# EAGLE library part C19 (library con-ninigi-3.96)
NINIGI
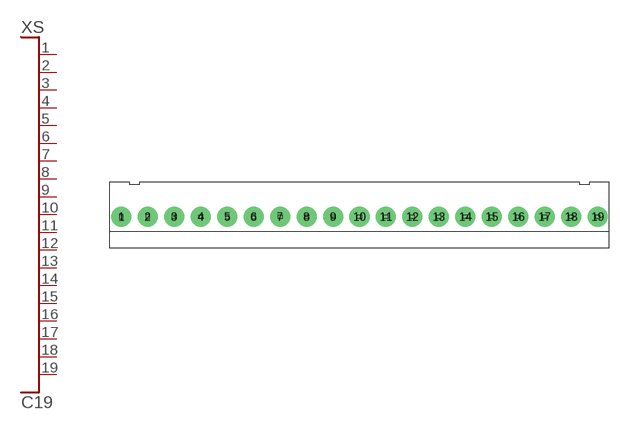
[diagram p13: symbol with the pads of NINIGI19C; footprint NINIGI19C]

Designator prefix XS

## C19  [NINIGI19C]
1  P$1
2  P$2
3  P$3
4  P$4
5  P$5
6  P$6
7  P$7
8  P$8
9  P$9
10  P$10
11  P$11
12  P$12
13  P$13
14  P$14
15  P$15
16  P$16
17  P$17
18  P$18
19  P$19

## Footprint NINIGI19C (pad centres in mm)
drill 1.6 pad 3: 1 -35.64,0; 2 -31.68,0; 3 -27.72,0; 4 -23.76,0; 5 -19.8,0; 6 -15.84,0; 7 -11.88,0; 8 -7.92,0; 9 -3.96,0; 10 0,0; 11 3.96,0; 12 7.92,0; 13 11.88,0; 14 15.84,0; 15 19.8,0; 16 23.76,0; 17 27.72,0; 18 31.68,0; 19 35.64,0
